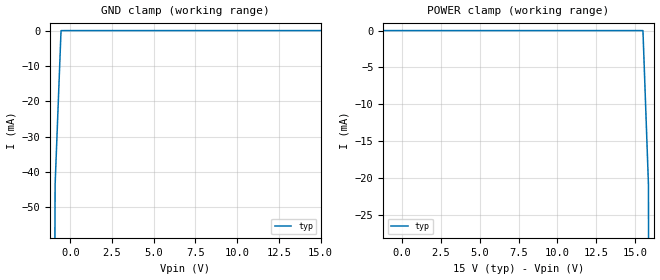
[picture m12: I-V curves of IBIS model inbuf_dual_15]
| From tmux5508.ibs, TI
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| inbuf_dual_15
[Model]   inbuf_dual_15
Model_type   Input
Vinl = 0.7
Vinh = 1.2
|   typ   min   max
C_comp   1.008417e-12   NA   NA
[Voltage Range]   15   NA   NA
[Temperature Range]   27   NA   NA
[Power Clamp Reference]   15   NA   NA
[GND Clamp Reference]   0   NA   NA
[GND Clamp]
|   Voltage   I(typ)   I(min)   I(max)
-20V      -37.7A     NA         NA
-1.263V   -433.2mA   NA         NA
-909.1mV  -43.46mA   NA         NA
-555.6mV  -9.656uA   NA         NA
15V       242.9nA    NA         NA
[POWER Clamp]
|   Voltage   I(typ)   I(min)   I(max)
-5V       651.2nA    NA         NA
15.51V    -2.991uA   NA         NA
15.86V    -20.85mA   NA         NA
16.21V    -364.4mA   NA         NA
30V       -22.82A    NA         NA
